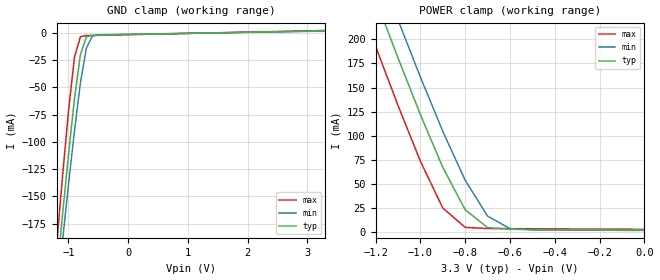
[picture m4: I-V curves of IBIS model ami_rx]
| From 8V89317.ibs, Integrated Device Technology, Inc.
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|   Model ami_rx
[Model]   ami_rx
Model_type   Input
Polarity   Non-Inverting
Enable   Active-High
C_comp   2.5000pF   2.4000pF   2.6000pF
Vinl=0.8V
Vinh=2.2V
[Temperature Range]   70.0000   0.1250k   0.0
[Voltage Range]   3.3000V   3.0000V   3.6000V
[GND_clamp]
|Voltage   I(typ)   I(min)   I(max)
-3.3V     -1.508A    -1.426A    -1.636A
-1.2V     -224.3mA   -244.1mA   -195.6mA
-1.1V     -167mA     -191mA     -132mA
-1V       -111.7mA   -139.4mA   -71.99mA
-900mV    -60.57mA   -90.15mA   -22.45mA
-800mV    -19.91mA   -45.96mA   -3.535mA
-700mV    -3.662mA   -13.89mA   -2.552mA
-600mV    -2.184mA   -3.02mA    -2.422mA
-400mV    -1.929mA   -1.733mA   -2.189mA
3.3V      1.821mA    1.591mA    2.124mA
[POWER_clamp]
|Voltage   I(typ)   I(min)   I(max)
-3.3V     1.612A     1.639A     1.58A
-1.3V     304.5mA    343.2mA    255.9mA
-1.2V     242mA      281.2mA    192.8mA
-1.1V     180.8mA    220.3mA    131.4mA
-1V       121.8mA    160.9mA    73.34mA
-900mV    66.92mA    104.4mA    24.66mA
-800mV    22.8mA     53.5mA     4.474mA
-700mV    4.271mA    16.21mA    3.307mA
-600mV    2.494mA    3.222mA    3.174mA
-500mV    2.33mA     1.848mA    3.057mA
0V        1.821mA    1.321mA    2.474mA
